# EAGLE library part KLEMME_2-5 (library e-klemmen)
Klemme 2 5
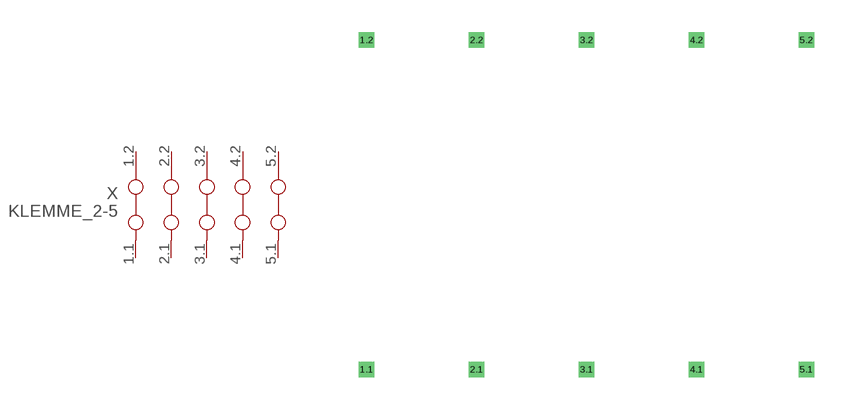
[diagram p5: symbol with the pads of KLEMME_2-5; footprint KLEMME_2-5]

Designator prefix X

## KLEMME_2-5  [KLEMME_2-5]
1.1  1.1  pas
1.2  1.2  pas
2.1  2.1  pas
2.2  2.2  pas
3.1  3.1  pas
3.2  3.2  pas
4.1  4.1  pas
4.2  4.2  pas
5.1  5.1  pas
5.2  5.2  pas

## Footprint KLEMME_2-5 (pad centres in mm)
Dummy
drill 0.2 pad 0.6 square: 1.1 0,-7.62; 1.2 0,7.62; 2.1 5.08,-7.62; 2.2 5.08,7.62; 3.1 10.16,-7.62; 3.2 10.16,7.62; 4.1 15.24,-7.62; 4.2 15.24,7.62; 5.1 20.32,-7.62; 5.2 20.32,7.62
